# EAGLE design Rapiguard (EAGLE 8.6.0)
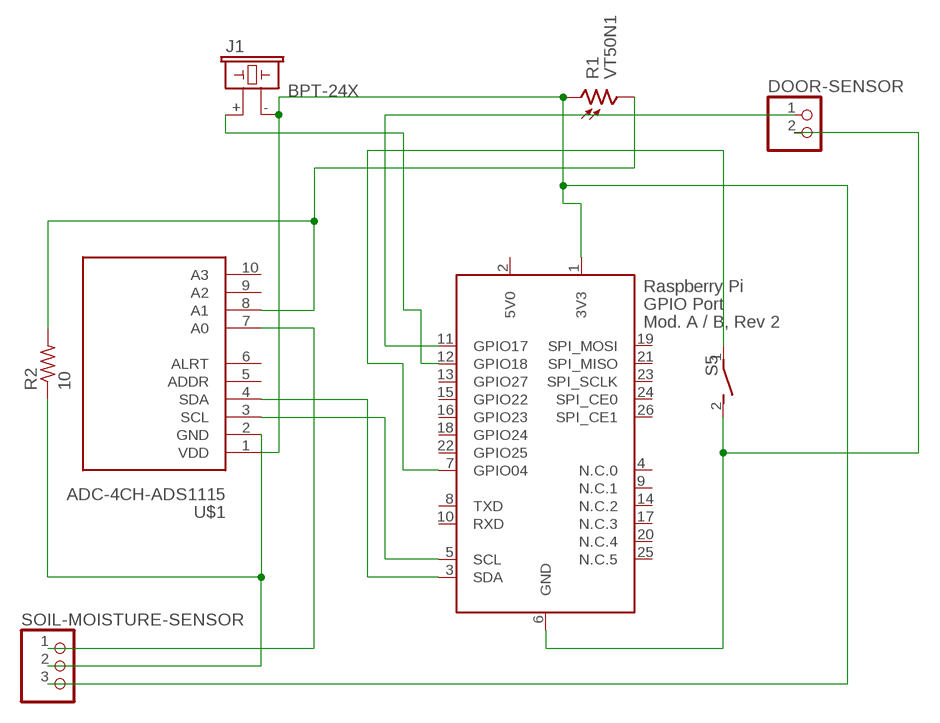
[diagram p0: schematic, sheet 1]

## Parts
DOOR-SENSOR  PINHD-1X2  [1X02]
J1  BPT-24X  [BPT-24X]
R1  VT50N1  [VT500]
R2  10  R-US_0204/7  [0204/7]
S5  SWITCH_01  [SWITCH_01]
SOIL-MOISTURE-SENSOR  PINHD-1X3  [1X03]
U$1  ADC-4CH-ADS1115  [ADC-4CH-ADS1115]
X2  RASPI_BOARD_B-_E0  [RASPI_BOARD_B-_EDGES_0DRILL]

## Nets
A0: SOIL-MOISTURE-SENSOR.1 U$1.7(A0)
GND: R2.1 SOIL-MOISTURE-SENSOR.2 U$1.2(GND)
GND_A: DOOR-SENSOR.2 S5.2 X2.6(GND)
GPIO04: S5.1 X2.7(GPIO04)
GPIO17: DOOR-SENSOR.1 X2.11(GPIO17)
GPIO18: J1.+ X2.12(GPIO18)
N$2: U$1.4(SDA) X2.3(SDA)
N$6: R1.2 R2.2 U$1.8(A1)
SCL: U$1.3(SCL) X2.5(SCL)
VCC: J1.- R1.1 SOIL-MOISTURE-SENSOR.3 U$1.1(VDD) X2.1(3V3)
Unconnected: U$1.5(ADDR) U$1.6(ALRT) U$1.9(A2) U$1.10(A3) X2.4(N.C.0) X2.8(TXD) X2.9(N.C.1) X2.10(RXD) X2.13(GPIO27) X2.14(N.C.2) X2.15(GPIO22) X2.16(GPIO23) X2.17(N.C.3) X2.18(GPIO24) X2.19(SPI_MOSI) X2.20(N.C.4) X2.21(SPI_MISO) X2.22(GPIO25) X2.23(SPI_SCLK) X2.24(SPI_CE0) X2.25(N.C.5) X2.26(SPI_CE1)

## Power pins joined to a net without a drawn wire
5V0: X2.2(5V0)

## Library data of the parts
DOOR-SENSOR = pinhead:PINHD-1X2: PIN HEADER
J1 = buzzer:BPT-24X; OC_FARNELL: unknown; OC_NEWARK: unknown
R1 = photo-elements:VT5*: Photoconductive Cell VT500 Sereis
R2 = resistor:R-US_: RESISTOR, American symbol
S5 = m-pad-2.1:SWITCH_01
SOIL-MOISTURE-SENSOR = pinhead:PINHD-1X3: PIN HEADER
U$1 = diy-modules:ADC-4CH-ADS1115: 4 Channel 16-Bit Analog-to-Digital Converter based on ADS1115 chip Arduino ADS1115 Getting Started Tutorial is available here: http://henrysbench.capnfatz.com/henrys-bench/arduino-voltage-measurements/arduino-ads1115-module-getting-started-tutorial/ ADS1115 datasheet is available here: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
X2 = raspberrypi_bastelstube_v13:RASPI_BOARD_B-: Raspberry Pi GPIO connector with markings for the outer dimensions of the Raspberry Pi board model B+ GPIO connector reduced to 26 pins to match models A and B with different sets of drill holes or mounting pads

## Module DOOR_SENSOR
Ports: 

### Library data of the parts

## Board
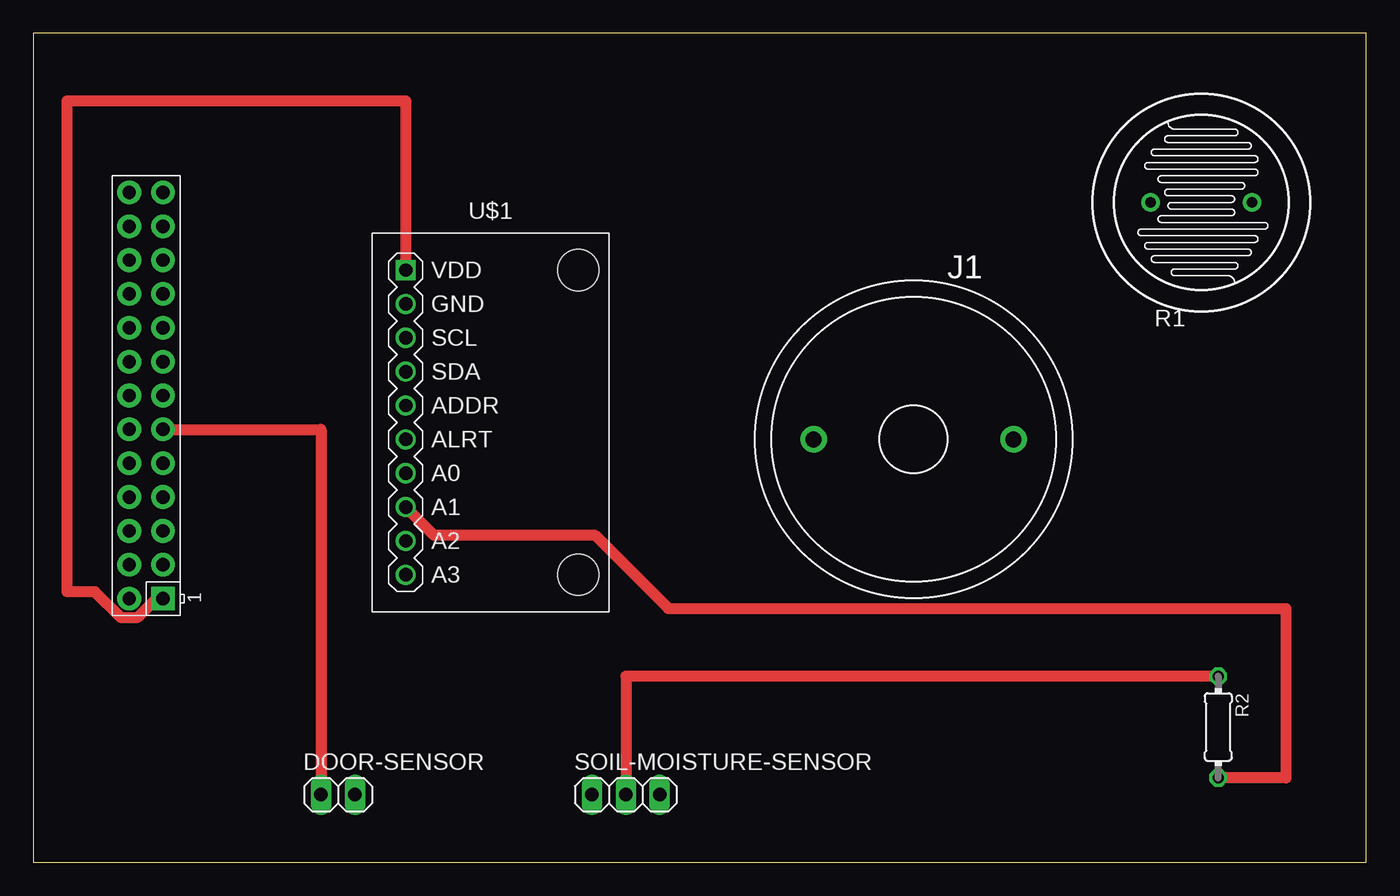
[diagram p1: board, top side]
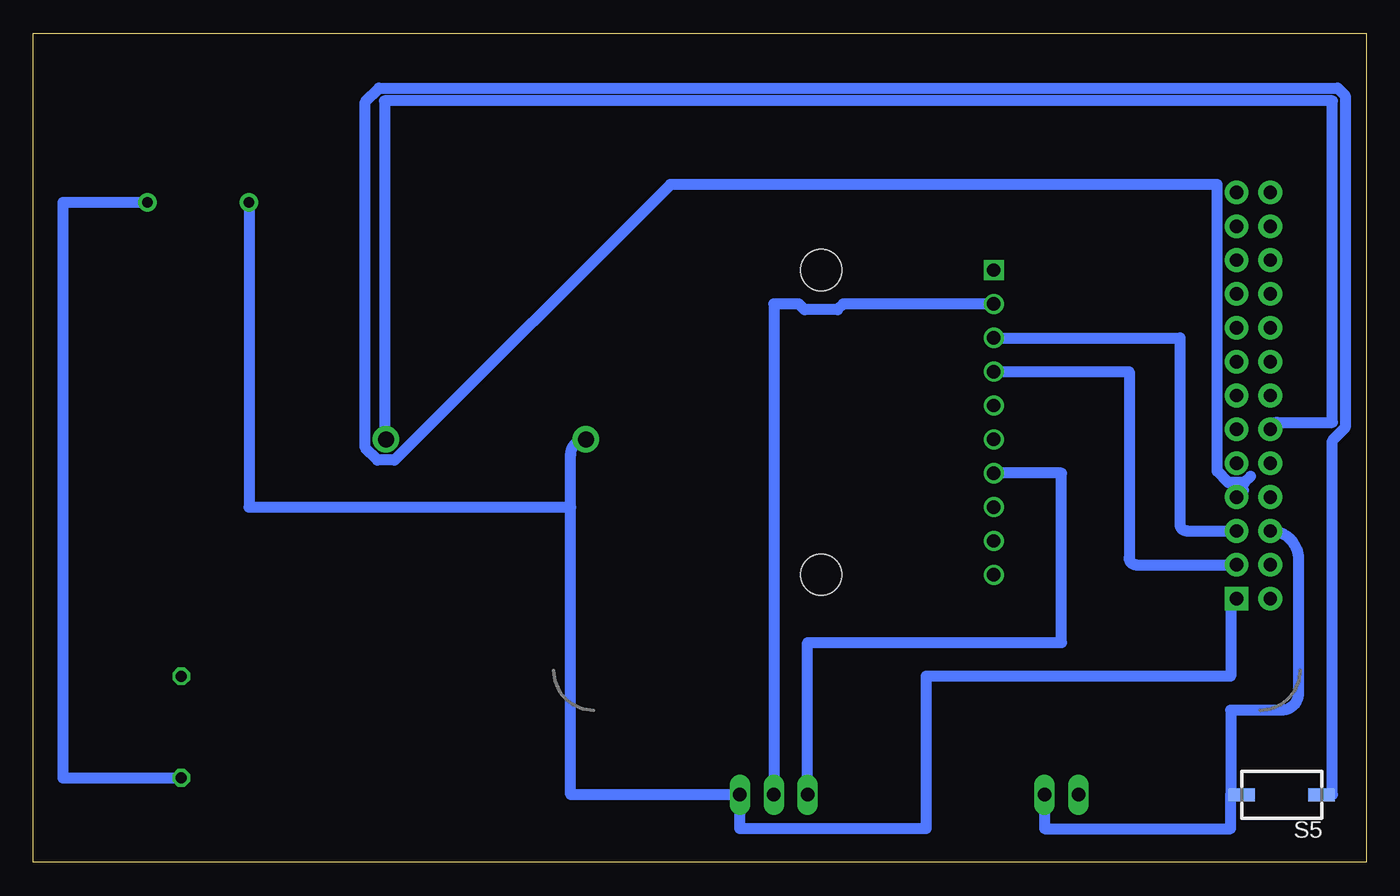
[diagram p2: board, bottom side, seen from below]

Size 100 x 62.22 mm. Coordinates in mm from the lower left corner, seen from the top.
Outline: 0,0 100,0 100,62.22 0,62.22 0,0
Copper layers (1*16): Top 0.035mm / dielectric 1.5mm / Bottom 0.035mm
Design rules "default": minimum track width 6mil, minimum drill 0.35mm, track to track 6mil, track to pad 6mil, pad to pad 6mil, via to via 6mil, smd to smd 6mil, copper to edge 40mil, drill to drill 6mil, minimum pad ring 10mil, minimum via ring 8mil, stop-mask expansion 4mil, vias tented up to drill 0mil, thermal gap 10mil

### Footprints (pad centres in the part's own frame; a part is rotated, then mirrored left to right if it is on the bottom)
1X02 = drill 1.016 long: 1 -1.27,0; 2 1.27,0
BPT-24X = drill 1.2 pad 2: + 7.5,0; - -7.5,0
VT500 = drill 0.8 pad 1.4: 1 -3.81,0; 2 3.81,0
0204/7 = drill 0.813 octagon: 1 -3.81,0; 2 3.81,0
SWITCH_01 = smd 2 x 1: 1 -3,0; 2 3,0
1X03 = drill 1.016 long: 1 -2.54,0; 2 0,0; 3 2.54,0
ADC-4CH-ADS1115 = drill 1 square: 1 -6.35,11.43 | drill 1: 2 -6.35,8.89; 3 -6.35,6.35; 4 -6.35,3.81; 5 -6.35,1.27; 6 -6.35,-1.27; 7 -6.35,-3.81; 8 -6.35,-6.35; 9 -6.35,-8.89; 10 -6.35,-11.43 | hole 3.1: 6.604,11.43; 6.604,-11.43
RASPI_BOARD_B-_EDGES_0DRILL = drill 1 pad 1.778 square: 1 8.37,51.23 | drill 1 pad 1.778: 2 8.37,53.77; 3 10.91,51.23; 4 10.91,53.77; 5 13.45,51.23; 6 13.45,53.77; 7 15.99,51.23; 8 15.99,53.77; 9 18.53,51.23; 10 18.53,53.77; 11 21.07,51.23; 12 21.07,53.77; 13 23.61,51.23; 14 23.61,53.77; 15 26.15,51.23; 16 26.15,53.77; 17 28.69,51.23; 18 28.69,53.77; 19 31.23,51.23; 20 31.23,53.77; 21 33.77,51.23; 22 33.77,53.77; 23 36.31,51.23; 24 36.31,53.77; 25 38.85,51.23; 26 38.85,53.77

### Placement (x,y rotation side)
DOOR-SENSOR  22.86,5.08 0 top
J1  66.04,31.75 0 top
R1  87.63,49.53 0 top
R2  88.9,10.16 270 top
S5  6.35,5.08 180 bottom
SOIL-MOISTURE-SENSOR  44.45,5.08 0 top
U$1  34.29,33.02 0 top
X2  60.96,11.43 90 top

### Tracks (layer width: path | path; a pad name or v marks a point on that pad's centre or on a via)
A0
  Bottom 0.813: SOIL-MOISTURE-SENSOR.1 41.91,16.51 22.86,16.51 22.86,29.21 U$1.7
GND
  Top 0.813: SOIL-MOISTURE-SENSOR.2 44.45,13.97 R2.1
  Bottom 0.813: U$1.2 39.23,41.91 39.66,41.48 42.12,41.48 42.56,41.91 44.45,41.91 SOIL-MOISTURE-SENSOR.2
GND_A
  Bottom 0.813: X2.6 arc90 5.08,22.77 5.08,12.7 arc90 6.35,11.43 10.16,11.43 10.16,5.08 | DOOR-SENSOR.2 24.13,2.54 10.16,2.54 10.16,5.08 | 8.89,5.08 S5.2 10.16,5.08
GPIO04
  Bottom 0.813: 9.21,27.94 arc-90 X2.7 9.73,27.91 9.13,28.51 | 3.81,5.08 S5.1 2.54,5.08 2.54,31.66 1.57,32.62 1.57,57.55 2.14,58.12 74.06,58.12 75.1,57.08 75.1,31.1 74.19,30.19 72.89,30.19 52.21,50.88 11.18,50.88 11.18,29.36 10.33,28.51 9.13,28.51 | 8.66,28.98 9.13,28.51
GPIO17
  Top 0.813: X2.11 21.59,32.5 DOOR-SENSOR.1
GPIO18
  Bottom 0.813: X2.12 arc90 6.67,33.02 2.54,33.02 2.54,57.15 73.66,57.15 73.66,31.75 J1.+
N$2
  Bottom 0.813: U$1.4 17.78,36.83 17.78,22.86 arc-90 17.26,22.34 X2.3
N$6
  Top 0.813: U$1.8 30.05,24.56 42.12,24.56 47.64,19.05 93.98,19.05 93.98,6.35 R2.2
  Bottom 0.813: R1.2 97.79,49.53 97.79,6.35 R2.2
SCL
  Bottom 0.813: U$1.3 13.97,39.37 13.97,25.4 arc-90 13.45,24.88 X2.5
VCC
  Top 0.813: X2.1 9.24,19.8 7.79,18.35 6.59,18.35 4.62,20.32 2.54,20.32 2.54,57.15 27.94,57.15 U$1.1
  Bottom 0.813: X2.1 arc-90 10.16,19.37 10.16,13.97 33.02,13.97 33.02,2.54 46.99,2.54 SOIL-MOISTURE-SENSOR.3 59.69,5.08 59.69,26.67 | 59.69,26.67 59.69,30.6 arc90 J1.- | R1.1 83.82,26.67 59.69,26.67

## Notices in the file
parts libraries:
diy-modules: Released under the Creative Commons Attribution 4.0 International License: http://creativecommons.org/licenses/by/4.0
m-pad-2.1: License : GNU General Public License version 2 (see bottom)
